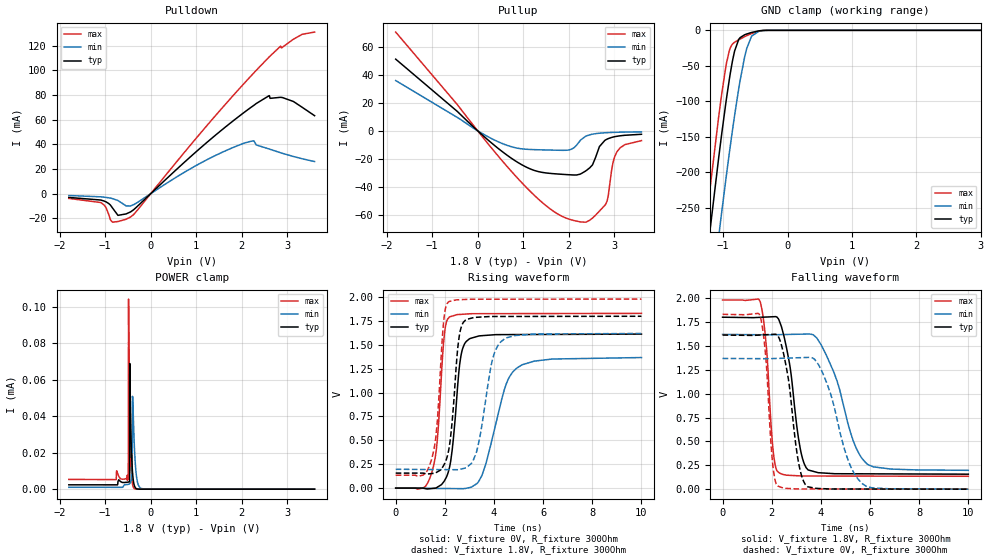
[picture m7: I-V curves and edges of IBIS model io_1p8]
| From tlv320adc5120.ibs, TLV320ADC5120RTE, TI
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|   io_1p8 Model
[Model]   io_1p8
Model_type   I/O
Polarity   Non-Inverting
Enable   Active-Low
Vinl = 0.63
Vinh = 1.17
Vmeas = 0.9
Vref = 0
Cref = 2pF
Rref = 100000
|   typ   min   max
C_comp   2.031pF   2.003pF   2.040pF
[Model spec]
|subparameter
Vinl   0.63   0.567   0.693
Vinh   1.17   1.053   1.287
| Where Nom  PVT is Nominal Process, 1.8V, 27C
|   Fast PVT is Strong Process,  1.98V, -40C
|   Slow PVT is Weak Process,   1.62V, 150C
[Voltage Range]   1.8   1.62   1.98
|Junction Temperature
[Temperature Range]   27   150   -40
[Pullup Reference]   1.8   1.62   1.98
[Pulldown Reference]   0   0   0
[Power Clamp Reference]   1.8   1.62   1.98
[GND Clamp Reference]   0   0   0
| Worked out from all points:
|   slope of the pulldown table from 0 to 0.27 V, typ, clamps not added: 28.7 ohm
|   slope of the pullup table from 0 to 0.27 V, typ, clamps not added: 34.9 ohm
|   GND clamp passes 1 mA (typ) near -0.46 V on its own axis
|   falling waveform, V_fixture 1.8V, R_fixture 300Ohm: 20-80 % time 512ps typ, 1.02ns min, 284ps max; typ from 1.8 V to 0.157 V
|   rising waveform, V_fixture 0V, R_fixture 300Ohm: 20-80 % time 343ps typ, 814ps min, 296ps max; typ from 0 V to 1.61 V
|   rising waveform, V_fixture 1.8V, R_fixture 300Ohm: 20-80 % time 317ps typ, 547ps min, 290ps max; typ from 0.157 V to 1.8 V
|   falling waveform, V_fixture 0V, R_fixture 300Ohm: 20-80 % time 478ps typ, 890ps min, 276ps max; typ from 1.61 V to 0 V
[Pulldown]
|   Voltage   I(typ)   I(min)   I(max)
-1.8V     -3.08mA    -1.517mA   -3.876mA
-1.098V   -5.187mA   -2.582mA   -7.205mA
-984.6mV  -6.638mA   -3.046mA   -11.24mA
-838.8mV  -11.7mA    -4.034mA   -23.14mA
-720mV    -17.6mA    -5.588mA   -22.59mA
-444.6mV  -14.83mA   -9.975mA   -18.98mA
894.6mV   30.58mA    20.65mA    40.32mA
1.823V    59.33mA    37.59mA    79.99mA
2.266V    71.56mA    42.73mA    97.86mA
2.601V    79.38mA    36.18mA    110.7mA
3.136V    74.65mA    30.08mA    125.2mA
3.6V      63.15mA    25.98mA    130.9mA
[GND Clamp]
|   Voltage   I(typ)   I(min)   I(max)
-1.8V     -772mA     -877.5mA   -717.3mA
-1.465V   -491.9mA   -601mA     -434.7mA
-1.233V   -304.2mA   -415.5mA   -245.5mA
-1.211V   -287.2mA   -398.7mA   -228.5mA
-1.071V   -180.6mA   -291.7mA   -122.8mA
-1.033V   -153.4mA   -263.9mA   -96.75mA
-898.2mV  -65.7mA    -168.9mA   -26.88mA
-822.6mV  -29.24mA   -120.1mA   -16.8mA
-666mV    -6.272mA   -37.4mA    -8.916mA
-558mV    -2.992mA   -8.162mA   -4.551mA
-390.6mV  -230.2uA   -452.8uA   -410.7uA
3.6V      0A         0A         0A
[Pullup]
|   Voltage   I(typ)   I(min)   I(max)
-1.8V     51.04mA    35.77mA    70.33mA
738mV     -19.52mA   -11.35mA   -28.79mA
1.267V    -28.52mA   -13.5mA    -46.69mA
1.872V    -31.09mA   -13.95mA   -61.27mA
2.266V    -30.75mA   -6.541mA   -65.01mA
2.52V     -24.5mA    -2.47mA    -62.38mA
2.59V     -19.16mA   -2.092mA   -60.23mA
2.677V    -11.28mA   -1.763mA   -57.27mA
2.844V    -5.993mA   -1.365mA   -50.13mA
2.974V    -4.527mA   -1.176mA   -22.89mA
3.06V     -3.951mA   -1.084mA   -15.11mA
3.6V      -2.518mA   -805.9uA   -7.051mA
[POWER Clamp]
|   Voltage   I(typ)   I(min)   I(max)
-1.8V     2.39uA     1.021uA    5.364uA
-493.2mV  3.889uA    2.624uA    6.047uA
-487.8mV  3.915uA    2.66uA     104.4uA
-466.2mV  4.151uA    2.929uA    47.82uA
-460.8mV  68.98uA    3.049uA    38.78uA
-433.8mV  29.58uA    4.479uA    12.69uA
-406.8mV  11.66uA    11.39uA    3.712uA
-401.4mV  9.599uA    50.99uA    2.862uA
-363.6mV  2.28uA     25.81uA    404.7nA
-309.6mV  228.5nA    6.403uA    6.342nA
-217.8mV  0A         443.4nA    0A
3.6V      0A         0A         0A
[Ramp]
R_load = 300
|   typ   min   max
dV/dt_r   0.967767/3.41047e-10   0.82044/8.14407e-10   1.09802/2.95662e-10
dV/dt_f   0.985782/5.09449e-10   0.853497/1.01139e-09   1.10707/2.83567e-10
[Falling Waveform]
V_fixture = 1.8V
V_fixture_min = 1.62V
V_fixture_max = 1.98V
R_fixture = 300Ohm
C_fixture = 0F
|   Time   V(typ)   V(min)   V(max)
0s        1.8V       1.62V      1.98V
1.531ns   1.799V     1.616V     1.961V
1.789ns   1.802V     1.616V     1.472V
2.063ns   1.805V     1.616V     392.2mV
2.288ns   1.775V     1.618V     173.8mV
3.168ns   414.2mV    1.622V     138.9mV
3.473ns   203.1mV    1.624V     137.6mV
4.228ns   167.1mV    1.4V       137.3mV
5.88ns    160.6mV    264.6mV    136.6mV
10ns      156.9mV    197.2mV    134.9mV
[Rising Waveform]
V_fixture = 0V
V_fixture_min = 0V
V_fixture_max = 0V
R_fixture = 300Ohm
C_fixture = 0F
|   Time   V(typ)   V(min)   V(max)
0s        3.015uV    142uV      641.4nV
1.462ns   -4.365mV   -3.067mV   158.4mV
1.683ns   8.079mV    -3.551mV   474.7mV
1.984ns   77.57mV    -4.211mV   1.616V
2.182ns   209.4mV    -4.646mV   1.791V
2.654ns   1.383V     -5.681mV   1.82V
2.983ns   1.56V      4.488mV    1.825V
3.511ns   1.597V     133.8mV    1.827V
4.911ns   1.608V     1.254V     1.828V
10ns      1.613V     1.368V     1.83V
[Rising Waveform]
V_fixture = 1.8V
V_fixture_min = 1.62V
V_fixture_max = 1.98V
R_fixture = 300Ohm
C_fixture = 0F
|   Time   V(typ)   V(min)   V(max)
0s        156.9mV    197.3mV    134.9mV
1.444ns   151.9mV    194.6mV    287.9mV
1.683ns   168.2mV    194.2mV    666.9mV
1.967ns   245.2mV    193.6mV    1.782V
2.147ns   386.2mV    193.3mV    1.95V
2.539ns   1.499V     192.6mV    1.972V
2.849ns   1.761V     211.5mV    1.976V
3.27ns    1.789V     363.3mV    1.978V
4.432ns   1.798V     1.564V     1.979V
10ns      1.8V       1.62V      1.98V
[Falling Waveform]
|Gnd
V_fixture = 0V
V_fixture_min = 0V
V_fixture_max = 0V
R_fixture = 300Ohm
C_fixture = 0F
|   Time   V(typ)   V(min)   V(max)
0s        1.613V     1.368V     1.83V
1.531ns   1.613V     1.366V     1.809V
1.771ns   1.617V     1.366V     1.34V
2.028ns   1.62V      1.367V     291mV
2.23ns    1.61V      1.369V     35.07mV
2.677ns   1.154V     1.372V     7.143mV
3.115ns   247mV      1.376V     2.186mV
3.449ns   27.14mV    1.379V     2.08mV
5.688ns   1.574mV    57.46mV    1.369mV
10ns      3.752uV    135.5uV    707.8nV
